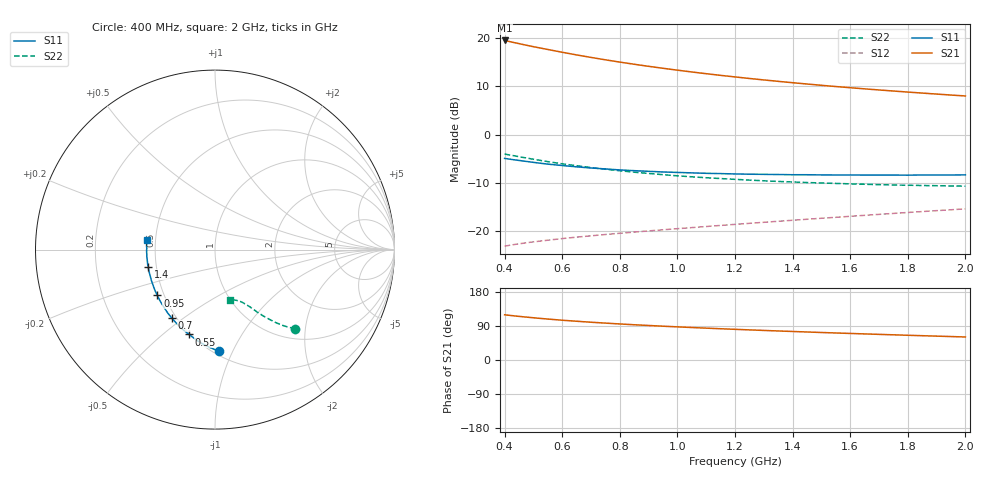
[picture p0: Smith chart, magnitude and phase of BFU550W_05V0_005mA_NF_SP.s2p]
! Filename:  P:\Prog\Test\Noise\ATS_data\Testdata_Net\06 Compressed Noise after Statistics\BFU550W_APM2013_11_D05_05p0V_005mA_NF_CM01_D.sf
! Date/Time: Tue 26/Mar/2013 16:25:22
! BFU550W_APM2013_11_D05_05p0V_1to35mA_NF_CM01_Bias4_R.sf
! Noise Parameter Data File
! BFU550W_APM2013_11_D05_05p0V_1to35mA_NF_CM01
! Date/time: Mon Mar 25 13:26:50 2013
! VAR V_out= 5.000000
! VAR I_out= 4.995000
! VAR V_in= 0.810900
! VAR I_in= 0.051405
! Device data file deembeded for feedlines and parallel
! Original file: \06 Compressed Noise after Statistics\BFU550W_APM2013_11_D05_05p0V_005mA_NF_CM01_R.sf
! Feed-files: PR019V01_070313_Feed1.s2p, PR019V01_070313_Feed2.s2p
! Parallel-file: PR019V01_070313_Par.s2p
# MHz S MA R 50
!  Freq-MHz  S11-mag  S11-arg  S21-mag  S21-arg  S12-mag  S12-arg  S22-mag  S22-arg
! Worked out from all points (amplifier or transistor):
!   37 points, 400 MHz to 2 GHz, reference 50 ohm
!   highest |S21| = 19.5 dB at 400 MHz (marker M1)
!   |S21| within 3 dB of that: start of sweep to 650.5 MHz
!   unconditionally stable (mu >= 1): 1.706 GHz to end of sweep
!   at 500 MHz: K = 0.52, MSG = 20.2 dB, |S12| = -22.2 dB
!   at 1.1 GHz: K = 0.87, MSG = 15.8 dB, |S12| = -19.0 dB
!   at 2 GHz: K = 1.02, MAG = 10.8 dB, |S12| = -15.4 dB
!   lowest NFmin = 0.56 dB at 420 MHz
!   S11 on the Smith chart (normalised r, x): 400 MHz: 0.53, -0.89; 550 MHz: 0.49, -0.62; 700 MHz: 0.47, -0.45; 950 MHz: 0.46, -0.28; 1.4 GHz: 0.45, -0.10; 2 GHz: 0.45, +0.05
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400  0.567 -87.5  9.417 119.3  0.07003 54.0  0.6287 -44.5
420  0.5555 -90.5  9.133 117.5  0.07174 53.5  0.613 -45.5
440  0.545 -93.3  8.865 115.9  0.07333 52.9  0.5977 -46.4
480  0.5252 -98.5  8.352 112.9  0.07622 52.1  0.5693 -48.1
500  0.5158 -101.2  8.117 111.4  0.07757 51.8  0.5559 -48.8
550  0.4946 -107.0  7.595 108.0  0.08075 51.2  0.525 -50.4
600  0.4785 -112.6  7.11 105.0  0.08387 50.8  0.4982 -51.7
650  0.4636 -117.5  6.671 102.3  0.08685 50.6  0.4765 -52.9
700  0.4511 -122.3  6.287 99.7  0.08965 50.5  0.4558 -54.0
750  0.4411 -126.5  5.936 97.3  0.09245 50.6  0.438 -54.9
800  0.4307 -130.7  5.624 95.1  0.09524 50.7  0.4226 -55.9
850  0.4231 -134.6  5.342 93.0  0.09795 50.9  0.4081 -56.5
950  0.4102 -141.5  4.853 89.2  0.1035 51.5  0.3846 -58.0
1050  0.4015 -147.7  4.444 85.7  0.109 52.2  0.3655 -59.3
1150  0.3947 -153.6  4.099 82.5  0.1148 52.8  0.3507 -60.6
1200  0.3915 -156.1  3.95 81.0  0.1177 53.1  0.3441 -61.3
1300  0.3876 -161.1  3.676 78.0  0.1237 53.8  0.3325 -62.5
1400  0.3842 -165.7  3.441 75.3  0.1298 54.4  0.3234 -63.7
1500  0.3825 -169.9  3.236 72.6  0.1362 54.9  0.3157 -65.2
1650  0.3809 -175.9  2.973 68.8  0.146 55.5  0.3062 -67.2
1750  0.3812 -179.3  2.823 66.5  0.1528 56.0  0.3007 -68.7
2000  0.383 172.3  2.51 60.8  0.1704 56.5  0.2924 -73.0
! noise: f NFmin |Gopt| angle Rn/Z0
400  0.5724  0.1598  45.6  0.0979
460  0.5769  0.1828  61.19  0.0896
600  0.6198  0.1769  56.1  0.1031
800  0.6398  0.1986  81.63  0.0917
1000  0.6828  0.2211  95.31  0.0874
1200  0.745  0.2376  109  0.0838
1400  0.7652  0.2679  127.4  0.0734
1600  0.8208  0.3135  143  0.0545
1800  0.8435  0.3529  157.4  0.0482
2000  0.8623  0.3647  172.5  0.049
